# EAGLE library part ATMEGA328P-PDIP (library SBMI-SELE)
Atmel 328P Through hole ATMEGA328P uC used in the Arduino 32kb flash, 1k EEPROM, 2k SRAM Datasheet SparkFun Products Storefront component: AVR 28 Pin 20MHz 32K 6A/D - ATMega328P (COM-09061) SparkFun Simon Says - Through-Hole Soldering Kit (KIT-10547) SparkFun Learn to Solder - Simon Says (KIT-13708) SparkFun BigTime Watch Kit (KIT-11734) SparkFun ClockIt (KIT-10930) SparkFun Serial Enabled LCD Kit (LCD-10097) SparkFun Simon Tilts - Through Hole Soldering Kit (KIT-12634) SparkFun Frequency Counter Kit (KIT-10140) FabFM Radio Kit (KIT-11043) SparkFun Binary Blaster Kit (KIT-12037) SparkFun Metro-Gnome (KIT-09236) ATmega328 with Arduino Optiboot (Uno) (DEV-10524)
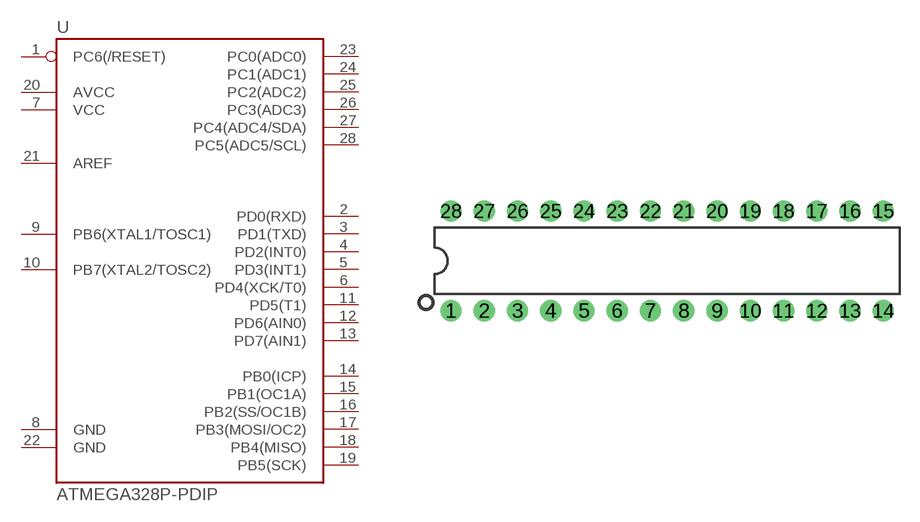
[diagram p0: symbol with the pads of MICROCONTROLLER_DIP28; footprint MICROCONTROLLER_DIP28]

Designator prefix U

## ATMEGA328P-PDIP (PROD_ID: IC-09136; VALUE: 328P)  [MICROCONTROLLER_DIP28]
1  PC6(/RESET)
2  PD0(RXD)
3  PD1(TXD)
4  PD2(INT0)
5  PD3(INT1)
6  PD4(XCK/T0)
7  VCC
8  GND
9  PB6(XTAL1/TOSC1)
10  PB7(XTAL2/TOSC2)
11  PD5(T1)
12  PD6(AIN0)
13  PD7(AIN1)
14  PB0(ICP)
15  PB1(OC1A)
16  PB2(SS/OC1B)
17  PB3(MOSI/OC2)
18  PB4(MISO)
19  PB5(SCK)
20  AVCC
21  AREF
22  GND
23  PC0(ADC0)
24  PC1(ADC1)
25  PC2(ADC2)
26  PC3(ADC3)
27  PC4(ADC4/SDA)
28  PC5(ADC5/SCL)

## Footprint MICROCONTROLLER_DIP28 (pad centres in mm)
Standard 28-pin DIP package. IC needs to have legs bent before insertion.
drill 0.813 pad 1.626: 1 -16.51,-3.81; 2 -13.97,-3.81; 3 -11.43,-3.81; 4 -8.89,-3.81; 5 -6.35,-3.81; 6 -3.81,-3.81; 7 -1.27,-3.81; 8 1.27,-3.81; 9 3.81,-3.81; 10 6.35,-3.81; 11 8.89,-3.81; 12 11.43,-3.81; 13 13.97,-3.81; 14 16.51,-3.81; 15 16.51,3.81; 16 13.97,3.81; 17 11.43,3.81; 18 8.89,3.81; 19 6.35,3.81; 20 3.81,3.81; 21 1.27,3.81; 22 -1.27,3.81; 23 -3.81,3.81; 24 -6.35,3.81; 25 -8.89,3.81; 26 -11.43,3.81; 27 -13.97,3.81; 28 -16.51,3.81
